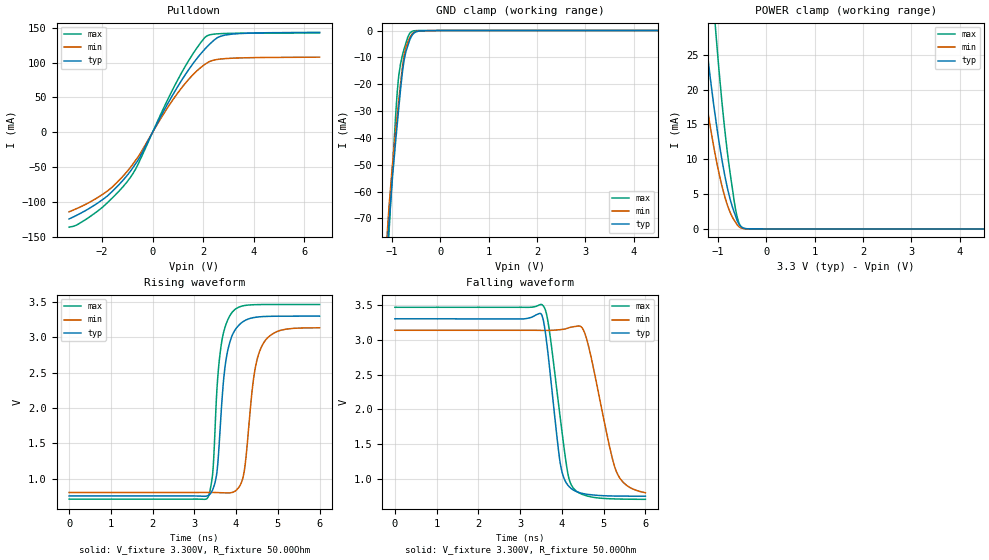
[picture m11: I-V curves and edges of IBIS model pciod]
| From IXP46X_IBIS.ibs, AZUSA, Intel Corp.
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[Model]   pciod
Model_type   I/O_open_drain
Vinl = 950.000mV
Vinh = 1.500V
Vmeas = 1.500V
Cref = 0.000F
|   typ   min   max
C_comp   3.000pF   2.700pF   3.300pF
[Voltage Range]   3.300V   3.135V   3.465V
[Temperature Range]   25.0   110.0   -40.0
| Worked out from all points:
|   slope of the pulldown table from 0 to 0.495 V, typ, clamps not added: 14.5 ohm
|   GND clamp passes 1 mA (typ) near -0.55 V on its own axis
|   POWER clamp passes 1 mA (typ) near -0.59 V on its own axis
|   falling waveform, V_fixture 3.300V, R_fixture 50.00Ohm: 20-80 % time 282ps typ, 491ps min, 346ps max; typ from 3.3 V to 0.753 V
|   rising waveform, V_fixture 3.300V, R_fixture 50.00Ohm: 20-80 % time 224ps typ, 265ps min, 188ps max; typ from 0.753 V to 3.3 V
[Pulldown]
|   Voltage   I(typ)   I(min)   I(max)
-3.3V     -124.6mA   -114.4mA   -136.4mA
-2.99V    -119.2mA   -109.6mA   -133.2mA
-1.995V   -97.34mA   -89.79mA   -108.3mA
-1.605V   -85.39mA   -79.22mA   -94.97mA
-895mV    -56.88mA   -51.41mA   -65.85mA
-525mV    -37.09mA   -32.82mA   -42.22mA
940mV     62.44mA    53.71mA    71.6mA
1.535V    95.49mA    80.32mA    109.3mA
2.08V     120mA      97.84mA    136.7mA
2.545V    135.5mA    104.5mA    141.4mA
2.89V     139.8mA    105.8mA    141.9mA
6.595V    143.5mA    107.9mA    142.6mA
[GND Clamp]
|   Voltage   I(typ)   I(min)   I(max)
-3.3V     -1.837A    -1.782A    -2.142A
-1.125V   -89.61mA   -82.47mA   -99.52mA
-1.065V   -72.55mA   -66.27mA   -76.21mA
-995mV    -55.6mA    -50.79mA   -53mA
-910mV    -38.32mA   -34.82mA   -27.37mA
-860mV    -28.72mA   -26.04mA   -16.73mA
-790mV    -16.24mA   -14.37mA   -9.578mA
-750mV    -11.01mA   -9.296mA   -6.858mA
-675mV    -5.744mA   -4.387mA   -2.48mA
-580mV    -1.627mA   -1.201mA   -252.6uA
0V        -56.89nA   -17.57nA   -32.79pA
6.595V    0A         0A         0A
[POWER Clamp]
|   Voltage   I(typ)   I(min)   I(max)
-3.3V     221.1mA    178.3mA    345.2mA
-1.48V    42.85mA    30.79mA    74.12mA
-1.43V    39.23mA    27.99mA    68.17mA
-1.265V   28.16mA    19.53mA    49.72mA
-1.065V   16.76mA    11.05mA    30.24mA
-1.025V   14.78mA    9.615mA    26.79mA
-915mV    9.907mA    6.159mA    18.18mA
-780mV    5.204mA    2.981mA    9.739mA
-635mV    1.89mA     986.7uA    2.845mA
-570mV    776uA      354.8uA    984.2uA
-515mV    310.8uA    129.8uA    274uA
6.595V    0A         0A         0A
[Ramp]
R_load = 50.00Ohm
|   typ   min   max
dV/dt_r   1.394uV/11.754ps   NA   56.121nV/9.008ps
dV/dt_f   1.528V/282.483ps   1.400V/490.759ps   1.654V/345.948ps
[Falling Waveform]
V_fixture = 3.300V
V_fixture_min = 3.135V
V_fixture_max = 3.465V
R_fixture = 50.00Ohm
|   Time   V(typ)   V(min)   V(max)
0s        3.3V       3.135V     3.465V
3.55ns    3.293V     3.133V     3.488V
3.69ns    2.678V     3.134V     3.171V
3.99ns    1.133V     3.146V     1.737V
4.18ns    886.8mV    3.173V     984.7mV
4.45ns    799.3mV    3.19V      789.3mV
4.64ns    778.1mV    2.903V     751.2mV
5.3ns     755.3mV    1.114V     713.5mV
5.55ns    754mV      908.8mV    710.5mV
6ns       753.2mV    802.4mV    708.3mV
[Rising Waveform]
V_fixture = 3.300V
V_fixture_min = 3.135V
V_fixture_max = 3.465V
R_fixture = 50.00Ohm
|   Time   V(typ)   V(min)   V(max)
0s        753.2mV    802.4mV    708.3mV
3.3ns     752.3mV    803.1mV    714.3mV
3.44ns    840.8mV    802.9mV    1.068V
3.64ns    1.906V     798.9mV    2.875V
3.77ns    2.718V     796.6mV    3.201V
3.97ns    3.099V     819mV      3.393V
4.19ns    3.23V      1.082V     3.449V
4.43ns    3.28V      2.458V     3.462V
4.63ns    3.293V     2.89V      3.464V
6ns       3.3V       3.135V     3.465V
